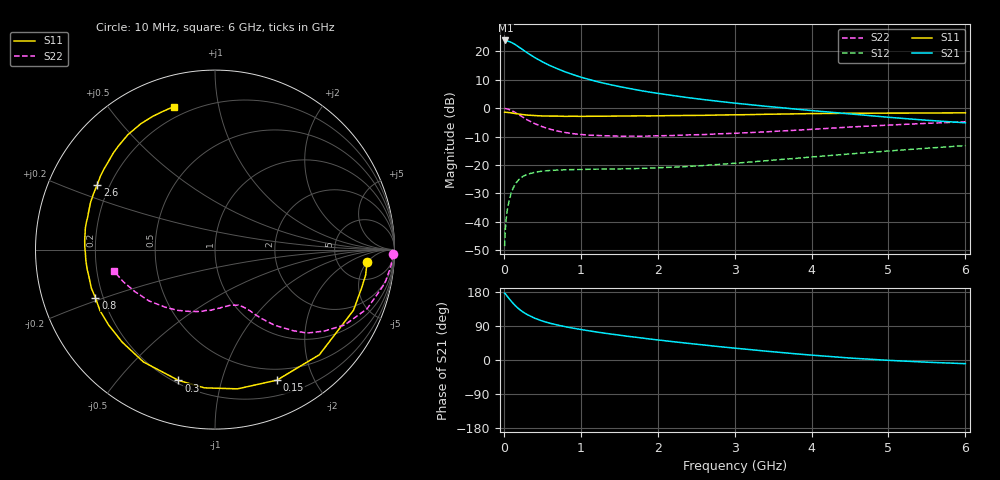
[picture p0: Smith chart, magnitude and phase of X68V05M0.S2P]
! SIEMENS Small Signal Semiconductors
! BFP193W
! Si NPN RF Bipolar Junction Transistor in SOT343
! VCE = 8 V  IC = 5 mA
! Common Emitter S-Parameters:  April 1994
# GHz  S  MA  R  50
!  f  S11  S21  S12  S22
! GHz  MAG  ANG  MAG  ANG  MAG  ANG  MAG  ANG
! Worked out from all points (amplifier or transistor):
!   40 points, 10 MHz to 6 GHz, reference 50 ohm
!   highest |S21| = 23.9 dB at 20 MHz (marker M1)
!   |S21| within 3 dB of that: start of sweep to 232.5 MHz
!   unconditionally stable (mu >= 1): 1.733 GHz to 4.345 GHz
!   at 200 MHz: K = 0.14, MSG = 23.2 dB, |S12| = -25.0 dB
!   at 1.5 GHz: K = 0.90, MSG = 14.5 dB, |S12| = -21.4 dB
!   at 6 GHz: K = 0.91, MSG = 4.0 dB, |S12| = -13.2 dB
!   lowest NFmin = 1.20 dB at 450 MHz
!   S11 on the Smith chart (normalised r, x): 10 MHz: 10, -5; 150 MHz: 0.37, -1.52; 300 MHz: 0.22, -0.74; 800 MHz: 0.17, -0.19; 2.6 GHz: 0.15, +0.25; 6 GHz: 0.15, +0.74
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0.01  0.8502 -4.7  15.56 176.3  0.0037 87.4  0.9915 -1.5
0.02  0.8512 -9.5  15.64 174.5  0.0074 83.9  0.986 -4.7
0.05  0.8425 -23.6  15.3 166.6  0.0182 77.8  0.9643 -11.3
0.1  0.8254 -45.2  14.4 154.2  0.034 67.0  0.9096 -21.2
0.15  0.8051 -64.6  13.21 143.0  0.0468 57.7  0.8363 -30.1
0.2  0.7859 -80.8  11.85 134.0  0.0561 50.2  0.7596 -36.7
0.25  0.7725 -94.4  10.68 126.5  0.0632 44.4  0.6921 -42.2
0.3  0.7566 -105.6  9.555 120.2  0.0679 39.5  0.6284 -46.0
0.4  0.7423 -122.5  7.844 110.4  0.0742 32.9  0.536 -51.8
0.5  0.7302 -135.1  6.583 102.9  0.0778 28.7  0.4721 -55.4
0.6  0.7264 -144.5  5.638 97.0  0.0799 25.9  0.4266 -58.2
0.8  0.7186 -157.9  4.359 87.8  0.0822 22.9  0.3727 -62.0
1  0.7184 -167.4  3.528 80.6  0.0831 21.8  0.3443 -65.7
1.1  0.7206 -171.4  3.24 77.2  0.0838 21.8  0.3353 -67.2
1.3  0.7224 -178.4  2.759 71.1  0.0844 22.2  0.3271 -71.0
1.6  0.7293 173.1  2.271 62.8  0.0858 24.3  0.3216 -76.7
2.2  0.7417 159.2  1.671 48.4  0.0914 29.7  0.3303 -89.5
2.6  0.7492 151.1  1.419 39.6  0.0979 33.9  0.3428 -98.6
3.2  0.7707 140.2  1.155 27.5  0.1126 38.4  0.3719 -112.1
4.5  0.8141 120.4  0.794 5.2  0.1564 41.0  0.4656 -142.1
5.5  0.8227 110.8  0.613 -5.8  0.1972 38.1  0.5411 -160.6
6  0.8293 106.0  0.553 -9.7  0.2192 36.1  0.5762 -168.1
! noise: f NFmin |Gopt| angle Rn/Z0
0.45  1.2  0.26  102  0.14
0.9  1.25  0.38  145  0.12
1.8  2.05  0.56  -161  0.12
